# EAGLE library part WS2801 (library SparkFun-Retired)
WS2801 3 Channel Constant Current LED Driver with programmable PWM outputs. Datasheet: http://www.sparkfun.com/datasheets/Components/LED/WS2801.pdf RETIRED: IC-10297 (also, wrong cat)
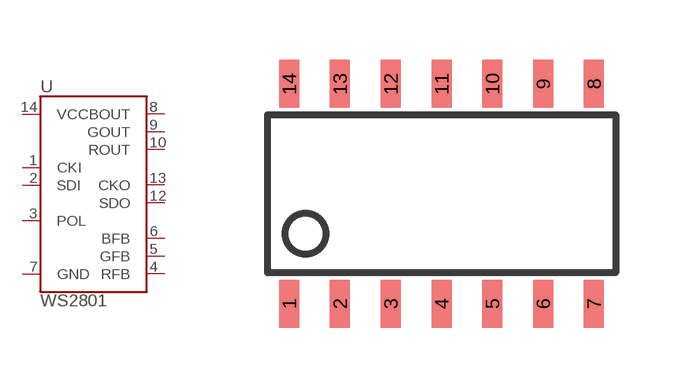
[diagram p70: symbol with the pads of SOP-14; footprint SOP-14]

Designator prefix U

## WS2801  [SOP-14]
1  CKI
2  SDI
3  POL
4  RFB
5  GFB
6  BFB
7  GND
8  BOUT
9  GOUT
10  ROUT
12  SDO
13  CKO
14  VCC

## Footprint SOP-14 (pad centres in mm)
14-pin SOP-14 package Used on WS2801 RGB controller
smd 0.5 x 1.2: 1 -3.81,-2.75; 2 -2.54,-2.75; 3 -1.27,-2.75; 4 0,-2.75; 5 1.27,-2.75; 6 2.54,-2.75; 7 3.81,-2.75; 8 3.81,2.75; 9 2.54,2.75; 10 1.27,2.75; 11 0,2.75; 12 -1.27,2.75; 13 -2.54,2.75; 14 -3.81,2.75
